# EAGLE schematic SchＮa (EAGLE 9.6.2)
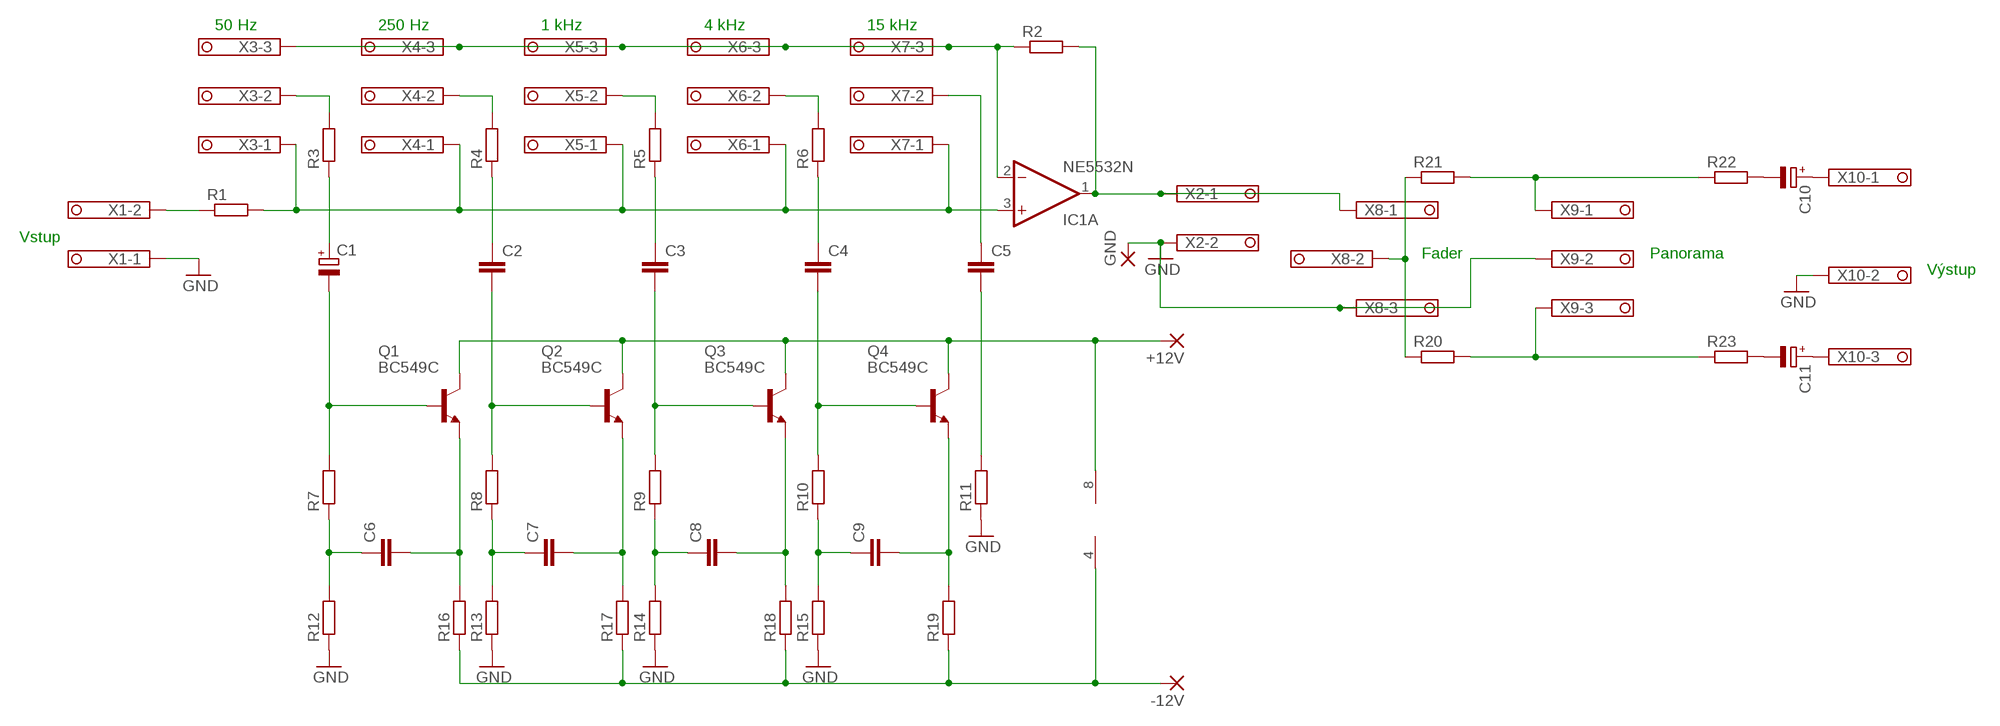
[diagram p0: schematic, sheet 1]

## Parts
+12V  1,6/0,8  [1,6/0,8]
-12V  1,6/0,8  [1,6/0,8]
C1  CPOL-EU153CLV-0605  [153CLV-0605]
C2  C-EUC1206  [C1206]
C3  C-EUC1206  [C1206]
C4  C-EUC1206  [C1206]
C5  C-EUC1206  [C1206]
C6  C-EU050-030X075  [C050-030X075]
C7  C-EUC1206  [C1206]
C8  C-EUC1206  [C1206]
C9  C-EUC1206  [C1206]
C10  CPOL-EU153CLV-0605  [153CLV-0605]
C11  CPOL-EU153CLV-0605  [153CLV-0605]
GND  1,6/0,8  [1,6/0,8]
IC1  NE5532N  [DIL08]
Q1  BC549C  [TO92-EBC]
Q2  BC549C  [TO92-EBC]
Q3  BC549C  [TO92-EBC]
Q4  BC549C  [TO92-EBC]
R1  R-EU_M1206  [M1206]
R2  R-EU_M1206  [M1206]
R3  R-EU_M1206  [M1206]
R4  R-EU_M1206  [M1206]
R5  R-EU_M1206  [M1206]
R6  R-EU_M1206  [M1206]
R7  R-EU_M1206  [M1206]
R8  R-EU_M1206  [M1206]
R9  R-EU_M1206  [M1206]
R10  R-EU_M1206  [M1206]
R11  R-EU_M1206  [M1206]
R12  R-EU_M1206  [M1206]
R13  R-EU_M1206  [M1206]
R14  R-EU_M1206  [M1206]
R15  R-EU_M1206  [M1206]
R16  R-EU_M1206  [M1206]
R17  R-EU_M1206  [M1206]
R18  R-EU_M1206  [M1206]
R19  R-EU_M1206  [M1206]
R20  R-EU_R1206  [R1206]
R21  R-EU_R1206  [R1206]
R22  R-EU_R1206  [R1206]
R23  R-EU_R1206  [R1206]
X1  1751248  [1751248]
X2  1751248  [1751248]
X3  1751251  [1751251]
X4  1751251  [1751251]
X5  1751251  [1751251]
X6  1751251  [1751251]
X7  1751251  [1751251]
X8  1751251  [1751251]
X9  1751251  [1751251]
X10  1751251  [1751251]

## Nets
GND: GND.1(P) R11.1 R12.1 R13.1 R14.1 R15.1 X1.1 X2.2 X8.3 X9.2 X10.2
N$1: IC1.1(A:OUT) R2.2 X2.1 X8.1
N$2: R1.1 X1.2
N$3: IC1.3(A:+IN) R1.2 X3.1 X4.1 X5.1 X6.1 X7.1
N$4: IC1.2(A:-IN) R2.1 X3.3 X4.3 X5.3 X6.3 X7.3
N$5: R3.2 X3.2
N$6: R4.2 X4.2
N$7: R5.2 X5.2
N$8: R6.2 X6.2
N$9: C1.+ R3.1
N$10: C2.1 R4.1
N$11: C3.1 R5.1
N$12: C4.1 R6.1
N$13: C5.1 X7.2
N$14: C5.2 R11.2
N$15: C1.- Q1.B R7.2
N$16: C2.2 Q2.B R8.2
N$17: C3.2 Q3.B R9.2
N$18: C4.2 Q4.B R10.2
N$19: +12V.1(P) IC1.8(P:V+) Q1.C Q2.C Q3.C Q4.C
N$20: C6.1 R7.1 R12.2
N$21: C7.1 R8.1 R13.2
N$22: C8.1 R9.1 R14.2
N$23: C9.1 R10.1 R15.2
N$24: C9.2 Q4.E R19.2
N$25: C8.2 Q3.E R18.2
N$26: C7.2 Q2.E R17.2
N$27: C6.2 Q1.E R16.2
N$28: -12V.1(P) IC1.4(P:V-) R16.1 R17.1 R18.1 R19.1
N$29: R20.1 R21.1 X8.2
N$30: R21.2 R22.1 X9.1
N$31: R20.2 R23.1 X9.3
N$32: C11.- R23.2
N$33: C10.- R22.2
N$34: C10.+ X10.1
N$35: C11.+ X10.3
Unconnected: IC1.5(B:+IN) IC1.6(B:-IN) IC1.7(B:OUT)

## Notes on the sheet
- 50 Hz | 250 Hz | 1 kHz | 4 kHz | 15 kHz
- Vstup
- Fader | Panorama
- Výstup

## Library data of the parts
+12V -12V GND = wirepad:1,6/0,8: THROUGH-HOLE PAD
C1 C10 C11 = rcl:CPOL-EU: POLARIZED CAPACITOR, European symbol; SPICEPREFIX: C
C2-C9 = rcl:C-EU: CAPACITOR, European symbol; SPICEPREFIX: C
IC1 = linear:NE5532: AUDIO AMPLIFIER
Q1-Q4 = transistor-npn:BC549*: NPN Transistor
R1-R23 = rcl:R-EU_: RESISTOR, European symbol; SPICEPREFIX: R
X1 X2 = con-phoenix-350:1751248: MKDS 1/ 2-3,5 Printklemme; OC_FARNELL: unknown; OC_NEWARK: unknown
X3-X10 = con-phoenix-350:1751251: MKDS 1/ 3-3,5 Printklemme Nennstrom: 10 A Bemessungsspannung: 160 V Raster: 3,5 mm Polzahl: 3 Montageart: Löten Anschlussart: Schraubanschluss Anschlussrichtung vom Leiter zur Platine: 0° Source: http://eshop.phoenixcontact.com .. 1751251.pdf; OC_FARNELL: unknown; OC_NEWARK: unknown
